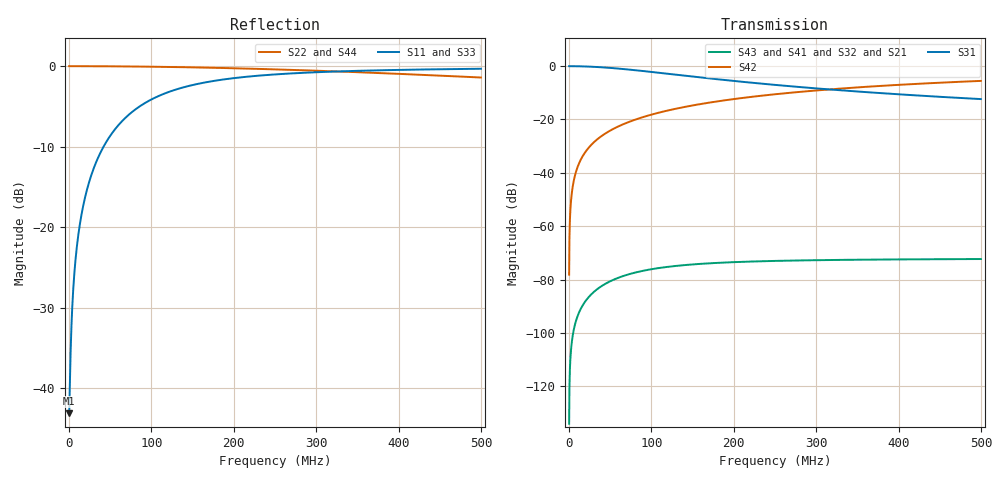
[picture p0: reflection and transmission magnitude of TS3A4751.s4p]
# GHz S MA R 50
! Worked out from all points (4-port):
!   2500 points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, 100 kHz to 499.9 MHz, reference 50 ohm
!   strongest paths, dB at 100 kHz, 125.1 MHz, 250.1 MHz, 375.1 MHz, 499.9 MHz:
!     S31: -0.1, -3.1, -7.1, -10.1, -12.4
!     S42: -78.1, -16.3, -10.6, -7.5, -5.6
!     S43: -133.9, -75.0, -73.0, -72.5, -72.3
!     S41: -133.9, -75.0, -73.0, -72.5, -72.3
!     S32: -133.9, -75.0, -73.0, -72.5, -72.3
!     S21: -133.9, -75.0, -73.0, -72.5, -72.3
!   lowest |S11| = -43.1 dB at 100 kHz (marker M1), VSWR 1.01, Z = 50.7 - j0.0813 ohm
!   |S11| at or under -10 dB: start of sweep to 41.87 MHz
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0.0001  0.006997 -6.6  2.01e-07 90.0  0.993 -0.0  2.01e-07 90.0
        2.01e-07 90.0  1 -0.0  2.01e-07 90.0  0.0001239 90.0
        0.993 -0.0  2.01e-07 90.0  0.006997 -6.6  2.01e-07 90.0
        2.01e-07 90.0  0.0001239 90.0  2.01e-07 90.0  1 -0.0
0.0041  0.03338 -79.9  8.235e-06 88.1  0.9925 -1.9  8.235e-06 88.1
        8.235e-06 88.1  1 -0.3  8.235e-06 88.1  0.005079 89.7
        0.9925 -1.9  8.235e-06 88.1  0.03338 -79.9  8.235e-06 88.1
        8.235e-06 88.1  0.005079 89.7  8.235e-06 88.1  1 -0.3
0.0131  0.104 -92.2  2.618e-05 84.0  0.9876 -6.0  2.618e-05 84.0
        2.618e-05 84.0  0.9999 -0.9  2.618e-05 84.0  0.01623 89.1
        0.9876 -6.0  2.618e-05 84.0  0.104 -92.2  2.618e-05 84.0
        2.618e-05 84.0  0.01623 89.1  2.618e-05 84.0  0.9999 -0.9
0.0341  0.2621 -103.8  6.61e-05 74.7  0.9579 -15.4  6.61e-05 74.7
        6.61e-05 74.7  0.9991 -2.4  6.61e-05 74.7  0.04221 87.6
        0.9579 -15.4  6.61e-05 74.7  0.2621 -103.8  6.61e-05 74.7
        6.61e-05 74.7  0.04221 87.6  6.61e-05 74.7  0.9991 -2.4
0.0693  0.4826 -118.3  0.0001217 60.9  0.8679 -29.3  0.0001217 60.9
        0.0001217 60.9  0.9963 -4.9  0.0001217 60.9  0.08553 85.1
        0.8679 -29.3  0.0001217 60.9  0.4826 -118.3  0.0001217 60.9
        0.0001217 60.9  0.08553 85.1  0.0001217 60.9  0.9963 -4.9
0.2223  0.8662 -150.5  0.0002185 29.3  0.4857 -61.4  0.0002185 29.3
        0.0002185 29.3  0.9641 -15.4  0.0002185 29.3  0.2655 74.6
        0.4857 -61.4  0.0002185 29.3  0.8662 -150.5  0.0002185 29.3
        0.0002185 29.3  0.2655 74.6  0.0002185 29.3  0.9641 -15.4
0.4999  0.9636 -165.9  0.0002431 13.9  0.2402 -77.6  0.0002431 13.9
        0.0002431 13.9  0.8503 -31.9  0.0002431 13.9  0.5263 58.1
        0.2402 -77.6  0.0002431 13.9  0.9636 -165.9  0.0002431 13.9
        0.0002431 13.9  0.5263 58.1  0.0002431 13.9  0.8503 -31.9
